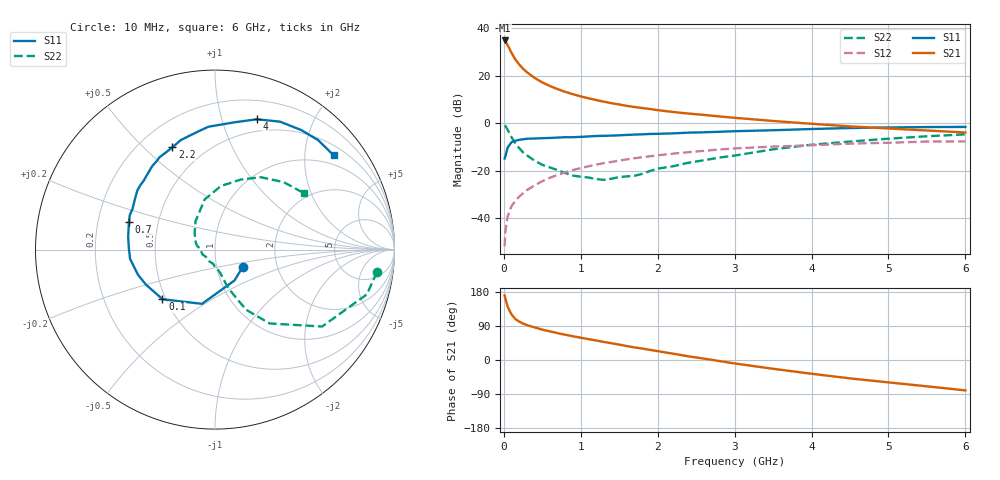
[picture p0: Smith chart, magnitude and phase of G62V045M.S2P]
! SIEMENS Small Signal Semiconductors
! BFG193
! Si NPN RF Bipolar Junction Transistor in SOT223
! VCE = 2 V  IC = 45 mA
! Common Emitter S-Parameters:  August  1996
# GHz  S  MA  R  50
!  f  S11  S21  S12  S22
! GHz  MAG  ANG  MAG  ANG  MAG  ANG  MAG  ANG
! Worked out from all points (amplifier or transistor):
!   36 points, 10 MHz to 6 GHz, reference 50 ohm
!   highest |S21| = 34.9 dB at 10 MHz (marker M1)
!   |S21| within 3 dB of that: start of sweep to 65.5 MHz
!   unconditionally stable (mu >= 1): 395.7 MHz to 2.566 GHz
!   at 250 MHz: K = 0.93, MSG = 26.2 dB, |S12| = -29.4 dB
!   at 1.4 GHz: K = 1.06, MAG = 10.9 dB, |S12| = -16.2 dB
!   at 6 GHz: K = 0.93, MSG = 1.9 dB, |S12| = -7.6 dB
!   S11 on the Smith chart (normalised r, x): 10 MHz: 1.33, -0.27; 100 MHz: 0.48, -0.32; 700 MHz: 0.34, +0.14; 2.2 GHz: 0.33, +0.61; 4 GHz: 0.38, +1.30; 6 GHz: 0.74, +2.69
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0.01  0.1821 -32.5  55.87 170.5  0.0026 87.2  0.911 -7.9
0.02  0.2035 -57.6  53.57 162.1  0.0054 80.8  0.8822 -16.4
0.05  0.3107 -103.5  44.39 140.2  0.0111 68.8  0.7347 -35.7
0.1  0.4026 -136.6  30.59 120.1  0.0181 65.2  0.5118 -53.5
0.15  0.4318 -153.3  22.18 108.0  0.0235 63.3  0.3789 -62.5
0.2  0.4518 -162.1  17.42 101.3  0.0287 65.7  0.3013 -66.0
0.25  0.4627 -168.7  14.16 96.0  0.0337 66.3  0.2455 -69.3
0.3  0.476 -173.8  11.97 92.1  0.0393 67.2  0.2127 -71.5
0.4  0.4806 178.4  9.088 86.0  0.0498 67.5  0.1642 -74.8
0.5  0.4885 171.8  7.295 80.1  0.0606 66.8  0.1343 -77.2
0.6  0.4943 167.1  6.12 75.5  0.0719 65.8  0.118 -80.8
0.7  0.5037 162.3  5.267 70.8  0.0825 64.5  0.104 -86.2
0.9  0.5124 153.7  4.115 62.6  0.1045 60.9  0.0795 -97.6
1.1  0.5315 146.4  3.381 55.1  0.125 57.1  0.0726 -116.7
1.6  0.5723 129.5  2.339 36.7  0.1753 46.0  0.0766 -168.0
2.2  0.6173 112.6  1.743 16.6  0.2311 32.0  0.1253 151.9
2.8  0.6673 97.4  1.405 -2.7  0.2823 17.6  0.1905 125.0
3.5  0.7183 81.1  1.126 -23.2  0.3254 0.0  0.2848 101.8
4  0.7625 72.2  0.983 -36.3  0.3472 -9.8  0.3559 84.7
4.5  0.7995 63.1  0.866 -48.5  0.3754 -19.9  0.4152 69.9
5.5  0.838 46.7  0.71 -69.5  0.4152 -42.9  0.5365 44.5
6  0.8444 38.4  0.644 -80.2  0.4183 -56.1  0.588 32.2
